ORGANIZATION_BLOCK MAIN:OB1
TITLE=Ascensore Didattico a 4 Piani
//Simulatore: 14
//Versione: 1.0
//Data: 08/03/2002

BEGIN
NETWORK 1 //Reset Merker al primo ciclo
//
LD SM0.1
S M0.0 1
R M0.1 1
R M1.0 3
R M2.0 5

NETWORK 2 //Legge Cella di Carico
//
LDN I0.4
MOVW AIW0 AC1

NETWORK 3 //Se il Peso supera 4 persone disabilita corsa
//
LDN I0.4
AW> AC1 +13000
S M2.0 1
NOT
R M2.0 1

NETWORK 4 //Allarme Sovracarico Cabina
//
LD M2.0
A SM0.5
= Q1.4

NETWORK 5 //Legge trasduttore posizine cabina
//
LD SM0.0
MOVW AIW2 AC2

NETWORK 6 //Setta Merker extracorsa
//
LDW>= AC2 +29100
OW<= AC2 +5500
S M2.1 1
NOT
R M2.1 1

NETWORK 7 //Carica valore impostazione temporizzatore da potenziometro analogico
//Se =0 imposta tempo minimo =20
LD SM0.0
MOVB SMB28 AC0
AB= AC0 0
MOVB 20 AC0

NETWORK 8 //Memorizza Movimento cabina in salita all'arresto
//
LDN I1.1
O M2.1
A Q0.0
S M2.2 1
R M2.3 1

NETWORK 9 //Memorizza Movimento cabina in Discesa all'arresto
//
LDN I1.1
O M2.1
A Q0.1
S M2.3 1
R M2.2 1

NETWORK 10 //Intervento pulsante di arresto cabina
//
LD Q0.0
O Q0.1
LDN I1.1
O M2.1
ALD
R Q0.0 2
S M0.0 1
R M0.1 1
S M2.4 1

NETWORK 11 //Reset Memoria Arresto
//
LD Q0.0
O Q0.1
R M2.4 1

NETWORK 12 //Temporizzazione richiusura porte
//
LDN M2.0
AN I1.7
O T32
TON T32 AC0

NETWORK 13 //Impostazione Merker Cabina libera
//
LDN Q0.0
AN Q0.1
A I0.4
= M0.0

NETWORK 14 //Tempo precedenza pulsanti cabina
//
LD T32
A I0.4
TON T33 AC0

NETWORK 15 //RESET Temporizzatori
//
LD T32
A T33
R T32 1

NETWORK 16 //Impostazione posizione cabina piano 1
//
//COMMENTI DEL SEGMENTO
//
LDN I0.0
S Q1.3 1
R Q1.0 3
MOVB 0 VB0

NETWORK 17 //Impostazione posizione cabina piano 2
//
//COMMENTI DEL SEGMENTO
//
LDN I0.1
S Q1.2 1
R Q1.3 1
R Q1.0 2
MOVB 1 VB0

NETWORK 18 //Impostazione posizione cabina piano 3
//
//COMMENTI DEL SEGMENTO
//
LDN I0.2
S Q1.1 1
R Q1.2 2
R Q1.0 1
MOVB 2 VB0

NETWORK 19 //Impostazione posizione cabina piano 4
//
//COMMENTI DEL SEGMENTO
//
LDN I0.3
S Q1.0 1
R Q1.1 3
MOVB 3 VB0

NETWORK 20 //Memorizzazione Chiamata/Mandata piano 1
//
LD I0.5
AN T32
LD I1.5
A M0.0
OLD
AN M0.1
S M0.1 1
MOVB 0 VB1

NETWORK 21 //Memorizzazione Chiamata/Mandata piano 2
//
LDN T32
A I0.6
LD M0.0
A I1.4
OLD
AN M0.1
S M0.1 1
MOVB 1 VB1

NETWORK 22 //Memorizzazione Chiamata/Mandata piano 3
//
LDN T32
A I0.7
LD M0.0
A I1.3
OLD
AN M0.1
S M0.1 1
MOVB 2 VB1

NETWORK 23 //Memorizzazione Chiamata/Mandata piano 4
//
LDN T32
A I1.0
LD M0.0
A I1.2
OLD
AN M0.1
S M0.1 1
MOVB 3 VB1

NETWORK 24 //Cabina arrivata al Piano
//
LD M0.1
LDB= VB1 0
AN I0.0
LDB= VB1 1
AN I0.1
OLD
LDB= VB1 2
AN I0.2
OLD
LDB= VB1 3
AN I0.3
OLD
ALD
S M1.0 1
R Q0.0 2

NETWORK 25 //Impostazioni Discesa cabina
//
LD M0.1
A M0.0
LDB> VB0 VB1
LDB= VB0 VB1
A M2.2
A M2.4
OLD
ALD
S Q0.1 1
R Q0.0 1

NETWORK 26 //Impostazioni Salita cabina
//
LD M0.1
A M0.0
LDB< VB0 VB1
LD M2.4
A M2.3
AB= VB0 VB1
OLD
ALD
S Q0.0 1
R Q0.1 1

NETWORK 27 //Apertura Porta cabuna
//
LDN I0.0
ON I0.1
ON I0.2
ON I0.3
A M1.0
AN M1.1
A I1.7
S Q0.3 1

NETWORK 28 //Impostazioni per apertura porta conclusa
//
LD M1.0
AN I1.7
R Q0.3 1
R M1.0 1
R M0.1 1

NETWORK 29 //Imposta richiusura porta
//
LD T32
S M1.1 1

NETWORK 30 //Comando chiusura porta
//
LD M1.1
AN M1.0
S Q0.2 1

NETWORK 31 //Intervento fotocellula sicurezza
//
LD M1.1
LD I1.6
O M2.0
ALD
S M1.0 1
R M1.1 1
R Q0.2 1
R T32 1

NETWORK 32 //RESET chiusura porta
//
LD M1.1
A I0.4
R Q0.2 1
R M1.1 1

NETWORK 33 //Gestione lampada piano 1
//
LD I0.0
A M0.1
A SM0.5
AB= VB1 0
ON I0.0
= Q0.4

NETWORK 34 //Gestione lampada piano 2
//
LD I0.1
A M0.1
A SM0.5
AB= VB1 1
ON I0.1
= Q0.5

NETWORK 35 //Gestione lampada piano 3
//
LD I0.2
A M0.1
A SM0.5
AB= VB1 2
ON I0.2
= Q0.6

NETWORK 36 //Gestione lampada piano 4
//
LD I0.3
A M0.1
A SM0.5
AB= VB1 3
ON I0.3
= Q0.7

NETWORK 37 //Segnalazione malfunzionamento
//
LD M2.1
A SM0.5
= Q1.5

END_ORGANIZATION_BLOCK

SUBROUTINE_BLOCK SBR_0:SBR0
TITLE=
//COMMENTI DEL SOTTOPROGRAMMA
//Premere F1 per visualizzare la guida e un esempio di programma
//

BEGIN
NETWORK 1 //TITOLO DEL SEGMENTO (una riga)
//
//COMMENTI DEL SEGMENTO
//

END_SUBROUTINE_BLOCK

